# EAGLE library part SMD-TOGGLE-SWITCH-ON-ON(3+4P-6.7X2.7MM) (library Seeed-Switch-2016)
311030001
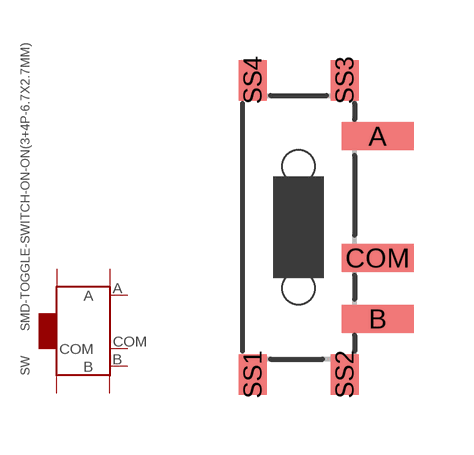
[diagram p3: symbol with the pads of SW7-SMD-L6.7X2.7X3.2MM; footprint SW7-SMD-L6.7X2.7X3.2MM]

Designator prefix SW

## SMD-TOGGLE-SWITCH-ON-ON(3+4P-6.7X2.7MM) (MPN: MK-12C02 G1.5; VALUE: MK-12C02 G1.5)  [SW7-SMD-L6.7X2.7X3.2MM]
A  A
B  B
COM  COM
SS1  SS1
SS2  SS2
SS3  SS3
SS4  SS4

## Footprint SW7-SMD-L6.7X2.7X3.2MM (pad centres in mm)
smd 1.8 x 0.7: A 1.978,2.286; B 1.978,-2.286; COM 1.978,-0.762
smd 0.7 x 1.016: SS1 -1.15,-3.683; SS2 1.15,-3.683; SS3 1.15,3.683; SS4 -1.15,3.683
hole 0.813 at 0,-1.524
hole 0.813 at 0,1.524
